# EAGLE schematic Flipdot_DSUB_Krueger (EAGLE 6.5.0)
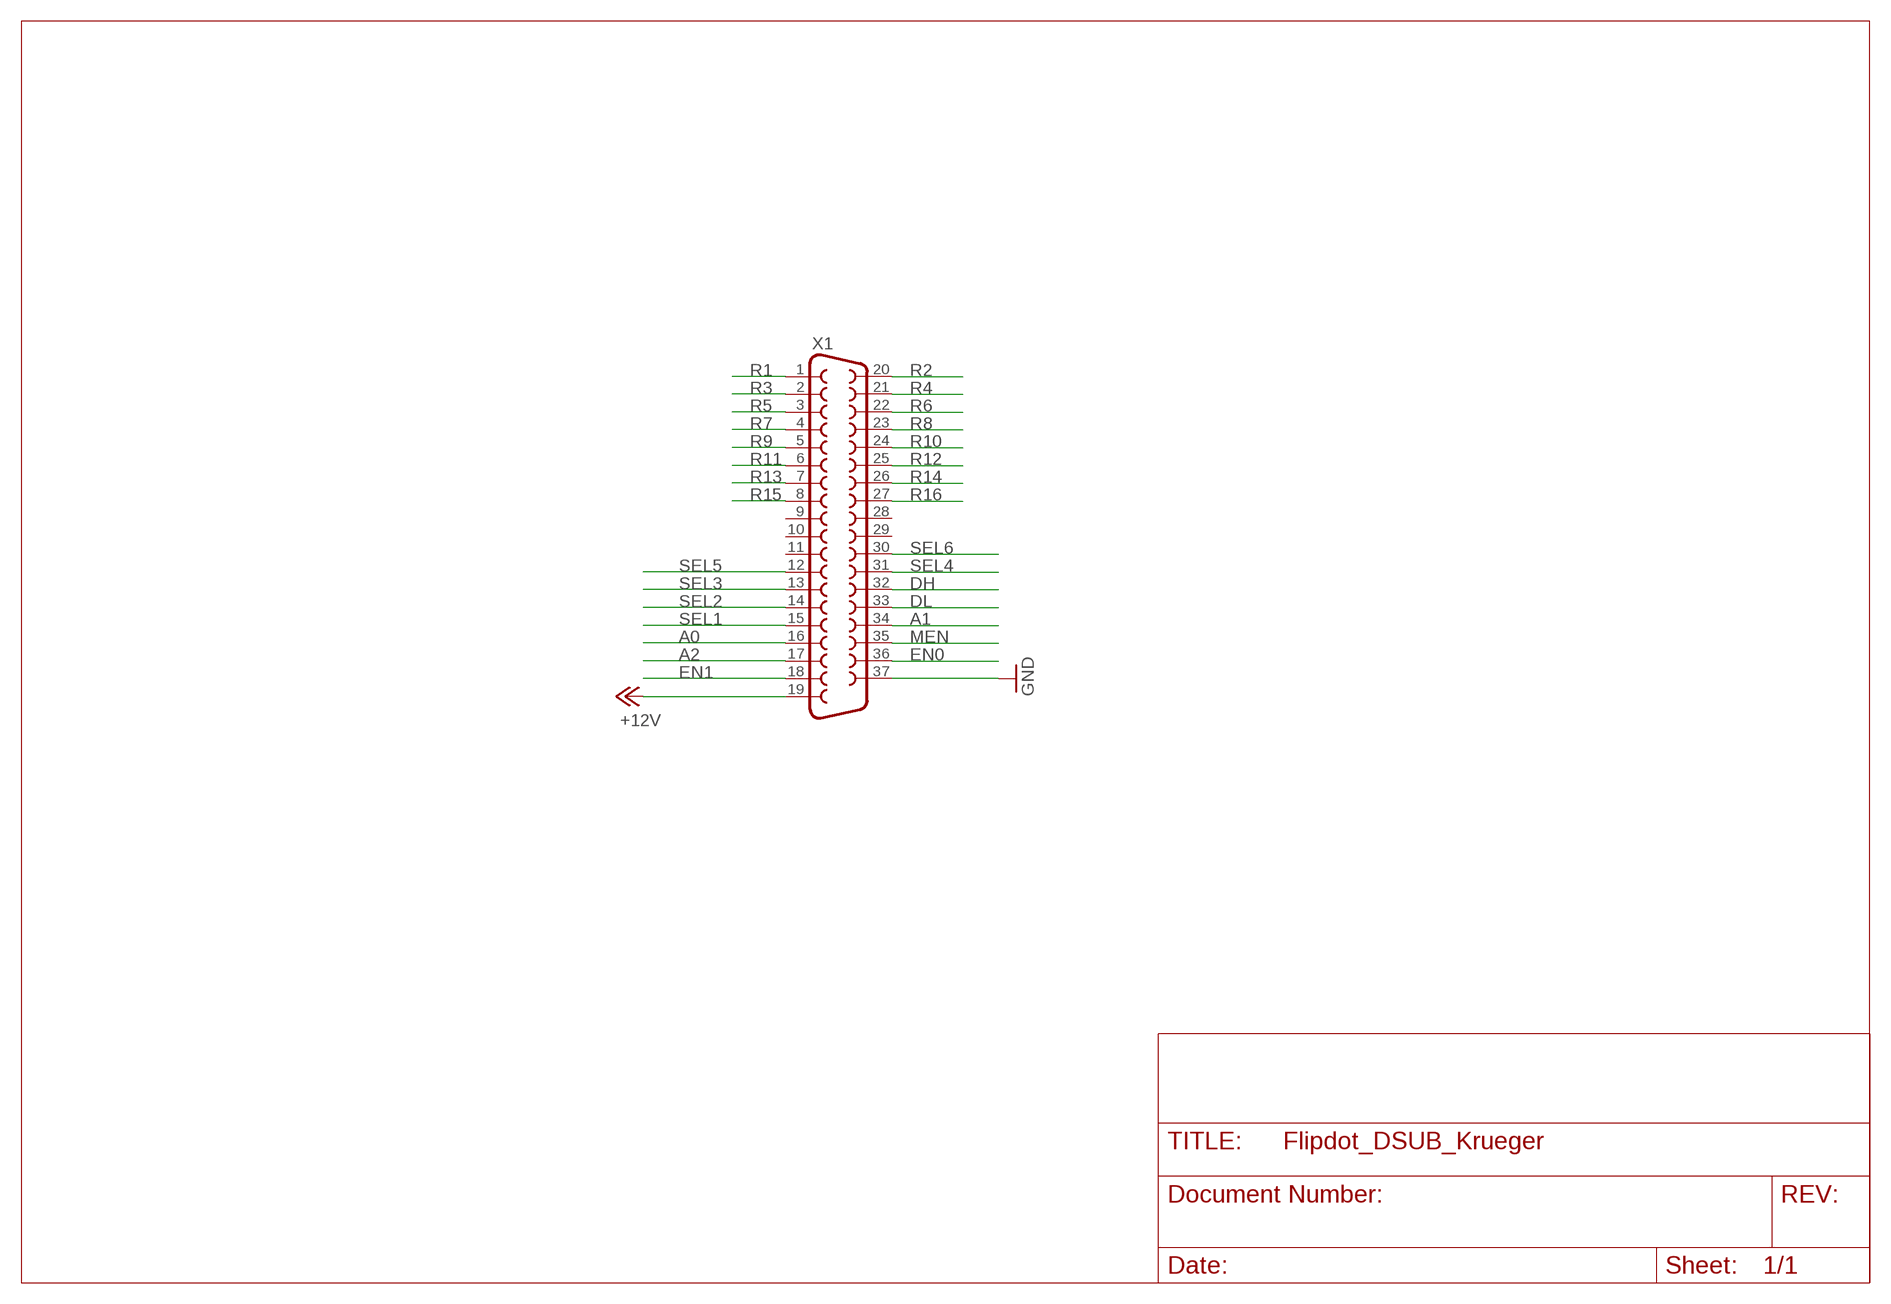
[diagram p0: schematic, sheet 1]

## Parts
X1  F37D  [F37D]

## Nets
+12V: X1.19
A0: X1.16
A1: X1.34
A2: X1.17
DH: X1.32
DL: X1.33
EN0: X1.36
EN1: X1.18
GND: X1.37
MEN: X1.35
R1: X1.1
R2: X1.20
R3: X1.2
R4: X1.21
R5: X1.3
R6: X1.22
R7: X1.4
R8: X1.23
R9: X1.5
R10: X1.24
R11: X1.6
R12: X1.25
R13: X1.7
R14: X1.26
R15: X1.8
R16: X1.27
SEL1: X1.15
SEL2: X1.14
SEL3: X1.13
SEL4: X1.31
SEL5: X1.12
SEL6: X1.30
Unconnected: X1.9 X1.10 X1.11 X1.28 X1.29

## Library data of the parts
X1 = con-subd:F37: SUB-D; OC_FARNELL: unknown; OC_NEWARK: unknown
